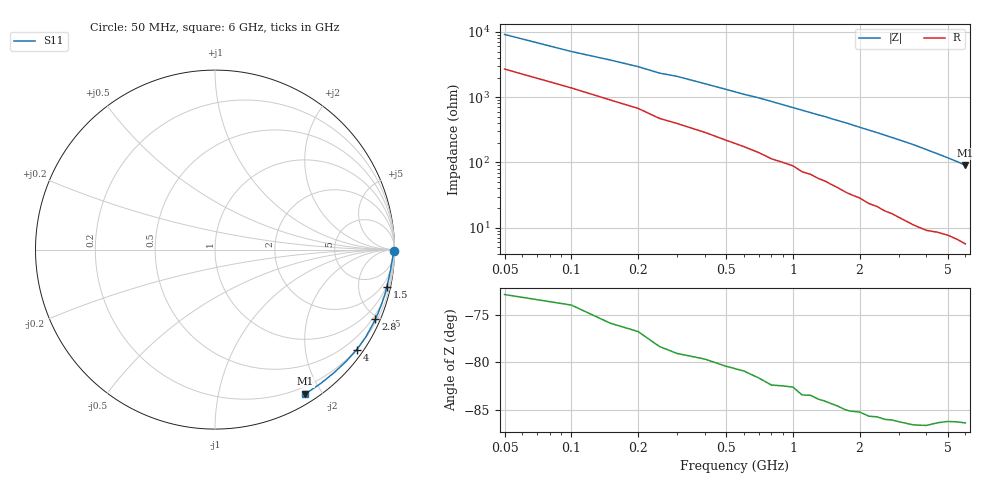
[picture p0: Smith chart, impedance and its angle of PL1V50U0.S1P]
! Infineon Technologies  Discrete & RF Semiconductors
! BAR 64-04W /-05W /-06W
! Si PIN Diode in SOT323
! VR = 1.5 V
! S-Parameters:  October  2008
# GHz  S  MA  R  50
!  f  S11
! GHz  MAG  ANG
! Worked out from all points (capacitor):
!   34 points, 50 MHz to 6 GHz, reference 50 ohm
!   read as one part to ground: C = 331 fF near 50 MHz
!   lowest |Z| = 90.3 ohm at 6 GHz (marker M1)
!   S11 on the Smith chart (normalised r, x): 50 MHz: open; 1.5 GHz: 0.91, -9.27; 2.8 GHz: 0.33, -4.81; 4 GHz: 0.18, -3.14; 6 GHz: 0.11, -1.80
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0.05  0.9968 -0.6
0.1  0.9945 -1.1
0.2  0.9922 -1.9
0.25  0.9914 -2.4
0.3  0.9909 -2.7
0.6  0.9859 -5.1
0.7  0.9853 -5.8
0.8  0.9848 -6.6
1  0.9817 -8.2
1.1  0.9822 -9.0
1.2  0.9808 -9.8
1.3  0.9805 -10.6
1.4  0.98 -11.3
1.5  0.9795 -12.2
1.6  0.9792 -13.0
1.8  0.9788 -14.6
2  0.9769 -16.4
2.2  0.9769 -18.1
2.4  0.9753 -19.8
2.6  0.9748 -21.6
2.8  0.9733 -23.4
3  0.9727 -25.2
3.5  0.971 -29.9
4  0.9671 -35.2
4.5  0.9599 -40.5
5  0.954 -46.0
5.5  0.9505 -51.7
6  0.9483 -57.9
